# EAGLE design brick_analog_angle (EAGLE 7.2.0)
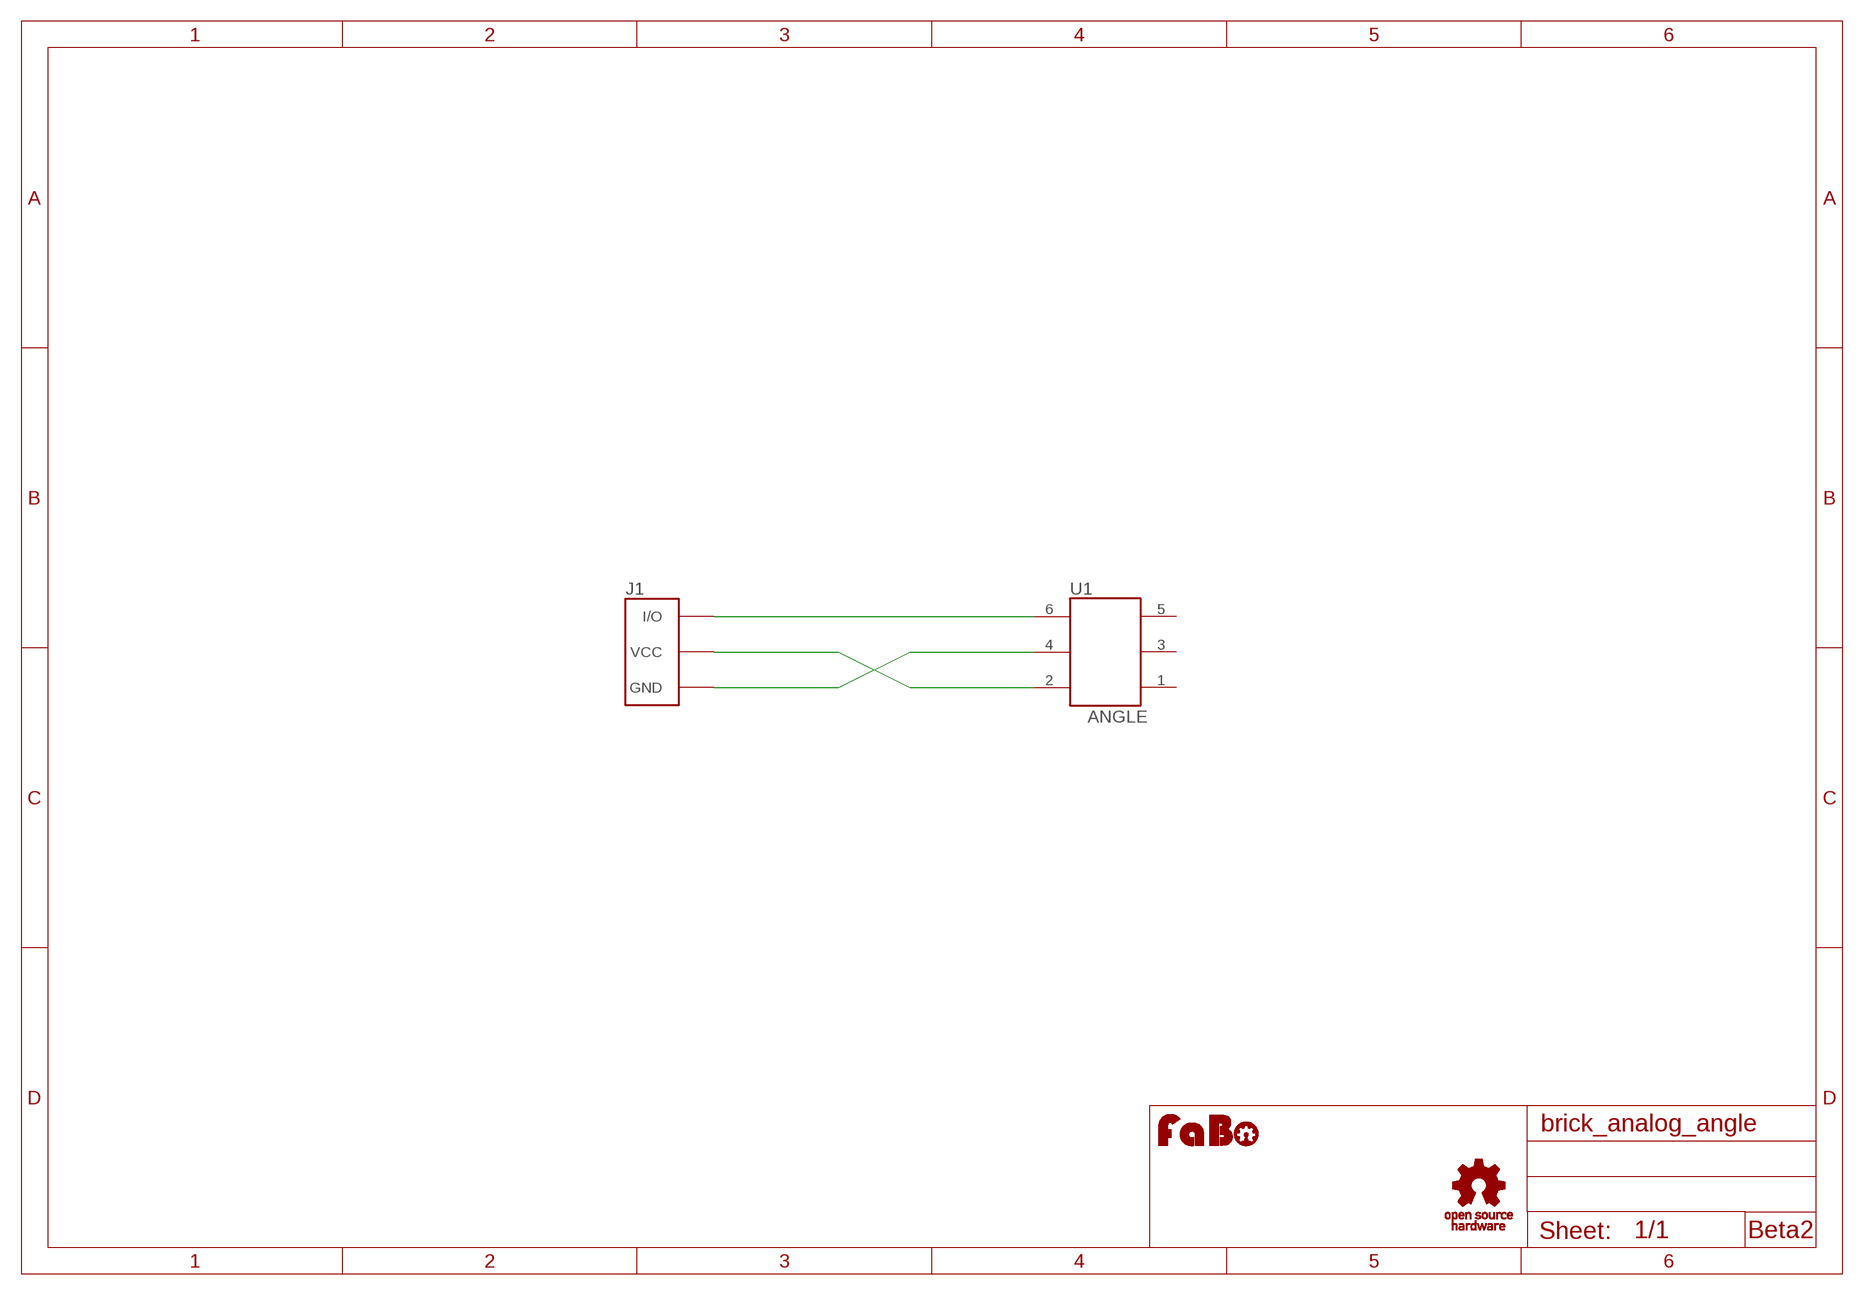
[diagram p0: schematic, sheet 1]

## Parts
J1  BRICK_3PIN  [BRICK_3PIN]
U1  ANGLE  ROTARYENCORDER_BRICK  [ROTARYENCORDER_BRICK]
U$2  LOGO_FABO-M  [LOGO_FABO_M]
U$5  LOGO_OSHW_T-M  [LOGO_OSHW_T_M]

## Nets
GND: J1.GND U1.4
N$1: J1.IN/OUT(I/O) U1.6
VCC: J1.VCC U1.2
Unconnected: U1.1 U1.3 U1.5

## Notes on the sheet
- Beta2

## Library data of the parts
J1 = gclue:BRICK_3PIN: FaBo Brick 3pin
U1 = gclue:ROTARYENCORDER_BRICK: Rotary Encorder for Brick
U$2 = FaBo:LOGO_FABO
U$5 = gclue:LOGO_OSHW_T

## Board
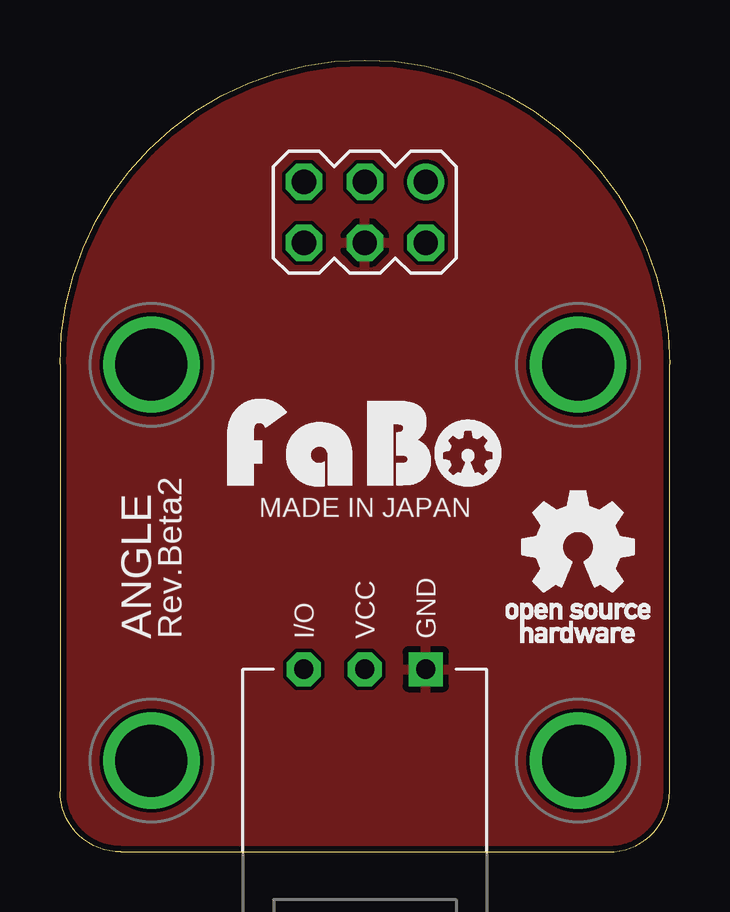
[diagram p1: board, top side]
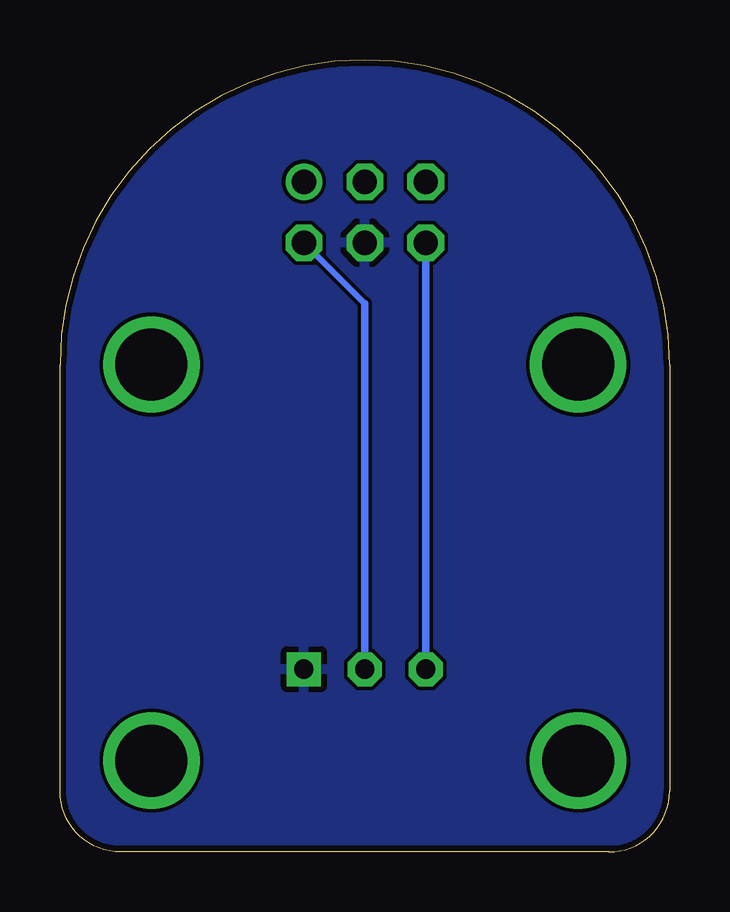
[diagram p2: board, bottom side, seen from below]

Size 25.4 x 33.02 mm. Coordinates in mm from the lower left corner, seen from the top.
Copper layers (1*16): Top 0.035mm / dielectric 1.5mm / Bottom 0.035mm
Design rules "Elecrow_2-layer_eagle_rule": minimum track width 6mil, minimum drill 12mil, track to track 6mil, track to pad 6mil, pad to pad 6mil, via to via 6mil, smd to smd 0mil, copper to edge 10mil, drill to drill 10mil, minimum pad ring 10mil, minimum via ring 6mil, stop-mask expansion 2mil, vias tented up to drill 100mil, thermal gap 10mil

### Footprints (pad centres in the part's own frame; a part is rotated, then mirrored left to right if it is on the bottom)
BRICK_3PIN = drill 0.8 pad 1.422 square: GND 2.54,-8.89 | drill 0.8 pad 1.422 octagon: IN/OUT -2.54,-8.89; VCC 0,-8.89 | drill 3 pad 3.81: P$5 -8.89,3.81; P$6 8.89,3.81; P$7 -8.89,-12.7; P$8 8.89,-12.7
ROTARYENCORDER_BRICK = drill 1.016: 1 -2.54,-1.27 | drill 1.016 octagon: 2 -2.54,1.27; 3 0,-1.27; 4 0,1.27; 5 2.54,-1.27; 6 2.54,1.27

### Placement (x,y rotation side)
J1  12.7,16.51 0 top
U1  12.7,26.67 180 top
U$2  12.7,15.24 0 top
U$5  21.59,12.7 0 top

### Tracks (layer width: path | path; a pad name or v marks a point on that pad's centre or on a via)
GND
  pour Bottom: -1.27,-1.27 26.67,-1.27 26.67,34.29 -1.27,34.29
  pour Top: -1.27,-1.27 26.67,-1.27 26.67,34.29 -1.27,34.29
N$1
  Bottom 0.305: U1.6 J1.IN/OUT
VCC
  Bottom 0.254: 12.7,22.86 U1.2
  Bottom 0.305: J1.VCC 12.7,22.86

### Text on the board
tPlace: MADE IN JAPAN | ANGLE | Rev.Beta2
